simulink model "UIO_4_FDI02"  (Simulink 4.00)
settings: Solver=VariableStepDiscrete  StartTime=0.0  StopTime=100  RelTol=1e-3
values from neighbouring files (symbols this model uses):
  A = [0.9944 -0.1203 -0.4302    [process_model02.m]
  Auio1 = F1    [UIO_KF_designs.m]
  Auio2 = F2    [UIO_KF_designs.m]
  B = [1 0    [process_model02.m]
  Buio1 = [T1*B K1]    [UIO_KF_designs.m]
  Buio2 = [T2*B K2]    [UIO_KF_designs.m]
  C = [1 0 0    [process_model02.m]
  Cuio1 = eye(3)    [UIO_KF_designs.m]
  Cuio2 = eye(3)    [UIO_KF_designs.m]
  D = zeros(2,2)    [process_model02.m]
  Duio1 = [zeros(3,2) H1]    [UIO_KF_designs.m]
  Duio2 = [zeros(3,2) H2]    [UIO_KF_designs.m]
  Ts = 0.1    [process_model02.m]
  x0 = [0.01 0.02 0.03]    [process_model02.m]
libraries: simulink3 x2

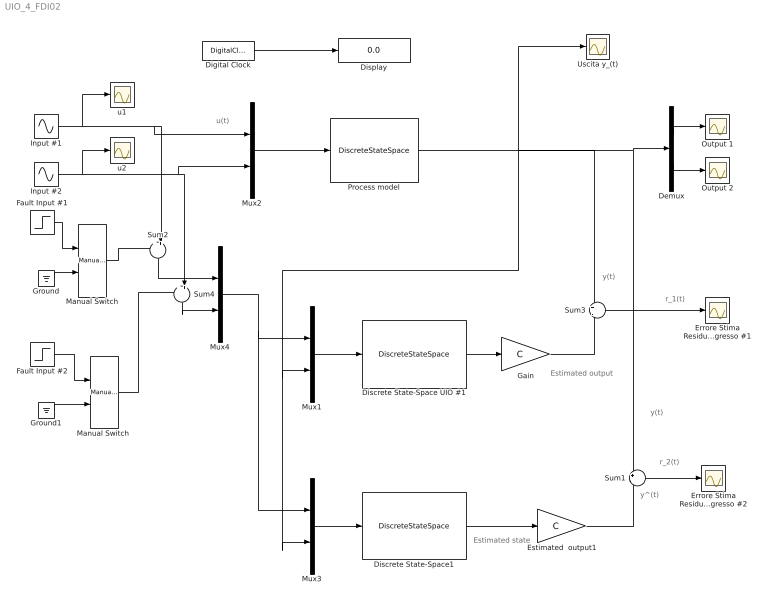
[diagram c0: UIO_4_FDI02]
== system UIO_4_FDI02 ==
  note: u(t)
  note: Estimated output
  note: y(t)
  note: Estimated state
  note: y^(t)
  note: y(t)
  note: r_1(t)
  note: r_2(t)
  Demux : Demux  Outputs=2  BusSelectionMode=off
  Digital Clock : DigitalClock  SampleTime=Ts
  Discrete State-Space UIO #1 : DiscreteStateSpace  A=Auio1  B=Buio1  C=Cuio1  D=Duio1  X0=0  SampleTime=Ts  Realization=auto
  Discrete State-Space1 : DiscreteStateSpace  A=Auio2  B=Buio2  C=Cuio2  D=Duio2  X0=0  SampleTime=Ts  Realization=auto
  Display : Display
  Errore Stima Residuo Ingresso #1 : Scope
  Errore Stima Residuo Ingresso #2 : Scope
  Estimated  output1 : Gain  Gain=C  Multiplication=Matrix(K*u)  SaturateOnIntegerOverflow=on
  Fault Input #1 : Step  Time=50  Before=0  After=1  SampleTime=Ts
  Fault Input #2 : Step  Time=50  Before=0  After=1  SampleTime=Ts
  Gain : Gain  Gain=C  Multiplication=Matrix(K*u)  SaturateOnIntegerOverflow=on
  Ground : Ground
  Ground1 : Ground
  Input #1 : Sin  SineType=Time-based  Amplitude=1  Bias=0  Frequency=1  Phase=0  Samples=10  SampleTime=Ts
  Input #2 : Sin  SineType=Time-based  Amplitude=0.5  Bias=0  Frequency=0.5  Phase=pi/2  Samples=10  SampleTime=Ts
  Manual Switch : simulink3/Nonlinear/Manual Switch  sw=0  action=0
  "Manual Switch " : simulink3/Nonlinear/Manual Switch  sw=0  action=0
  Mux{1..4} (4 alike) : Mux  Inputs=2
  Output 1 : Scope
  Output 2 : Scope
  Process model : DiscreteStateSpace  A=A  B=B  C=C  D=D  X0=x0  SampleTime=Ts  Realization=auto
  Sum1 : Sum  Inputs=+|-  SaturateOnIntegerOverflow=on
  Sum2 : Sum  Orientation=down  Inputs=++|  SaturateOnIntegerOverflow=on
  Sum3 : Sum  Inputs=+|-  SaturateOnIntegerOverflow=on
  Sum4 : Sum  Orientation=down  Inputs=++|  SaturateOnIntegerOverflow=on
  Uscita y_(t) : Scope
  u1 : Scope
  u2 : Scope
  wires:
  Digital Clock/1 -> Display/1
  Mux2/1 -> Process model/1
  Input #1/1 -> u1/1, Mux2/1, Sum2/2
  Process model/1 -> Uscita y_(t)/1, Mux1/2, Mux3/2, Sum3/1, Demux/1, Sum1/1
  Sum3/1 -> Errore Stima Residuo Ingresso #1/1
  Sum1/1 -> Errore Stima Residuo Ingresso #2/1
  Input #2/1 -> u2/1, Mux2/2, Sum4/2
  Ground/1 -> Manual Switch/2
  Fault Input #1/1 -> Manual Switch/1
  Ground1/1 -> "Manual Switch "/2
  Fault Input #2/1 -> "Manual Switch "/1
  "Manual Switch "/1 -> Sum4/1
  Demux/1 -> Output 1/1
  Demux/2 -> Output 2/1
  Manual Switch/1 -> Sum2/1
  Mux1/1 -> Discrete State-Space UIO #1/1
  Mux3/1 -> Discrete State-Space1/1
  Sum2/1 -> Mux4/1
  Sum4/1 -> Mux4/2
  Mux4/1 -> Mux1/1, Mux3/1
  Discrete State-Space UIO #1/1 -> Gain/1
  Gain/1 -> Sum3/2
  Estimated  output1/1 -> Sum1/2
  Discrete State-Space1/1 -> Estimated  output1/1
